(* 	
	Program Name: 	ACS_INITIALIZATION_WITH_BRAKE
	Purpose:		Example of Initialization of Drive with a Brake
	When Executed:	Enables drive and performs homing routine if there are no faults
*)
PROGRAM ACS_INITIALIZATION_WITH_BRAKE
VAR_IN_OUT
	Axis:ACS_DRIVE_TYPE;
END_VAR

//If there are faults or if the drive is enabled and homed, this should just fall through

//Only if there are no faults...
IF Axis.InputFaultActive < 1 THEN

	//If we are not enabled, then enable
	IF Axis.InputStatusDriveEnabled < 1 THEN
		ACS_CMD_ENABLE(Axis:=Axis);

	ELSE 
		//If we are enabled, but not homed, then home
		IF Axis.InputStatusDriveHomed < 1 THEN
			//Brake is turned off after a period of time while the drive is enabling - so we need to wait until we get a signal from the drive that the brake is off
			IF Axis.InputStatusDriveBrakeNotActive = 1 THEN
				ACS_CMD_HOME(Axis:=Axis);
			END_IF
		END_IF
	END_IF
	
END_IF

END_PROGRAM
